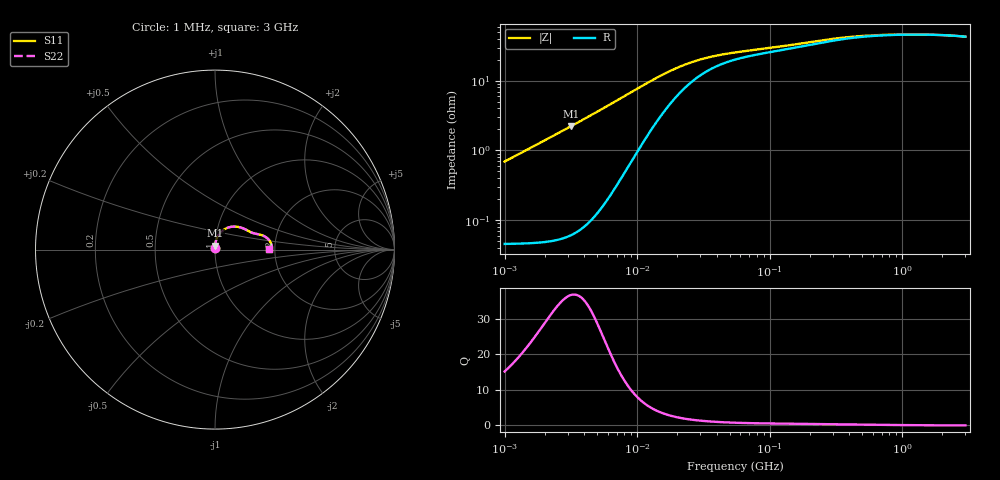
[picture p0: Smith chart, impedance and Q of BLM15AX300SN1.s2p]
! BLM15AX300SN1
# Hz S RI R 50
!Freq.(Hz) S11(Real) S11(Imag) S21(Real) S21(Imag) S12(Real) S12(Imag) S22(Real) S22(Imag)
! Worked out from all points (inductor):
!   401 points, 1 MHz to 3 GHz, reference 50 ohm
!   read as one part in series: L = 110 nH near 1.041 MHz
!   highest Q = 36.7 at 3.193 MHz (marker M1), where L = 112 nH
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1000000  0.000502 0.0069  0.9995 -0.0069  0.9995 -0.0069  0.000502 0.0069
1040844  0.000506 0.00718  0.9995 -0.00718  0.9995 -0.00718  0.000506 0.00718
1173660  0.000522 0.0081  0.9995 -0.0081  0.9995 -0.0081  0.000522 0.0081
3192880  0.00111 0.0224  0.9989 -0.0224  0.9989 -0.0224  0.00111 0.0224
3823119  0.00148 0.027  0.9985 -0.027  0.9985 -0.027  0.00148 0.027
5938264  0.00378 0.0429  0.9962 -0.0429  0.9962 -0.0429  0.00378 0.0429
8686058  0.0102 0.0643  0.9898 -0.0643  0.9898 -0.0643  0.0102 0.0643
1.172775e7  0.0228 0.0865  0.9772 -0.0865  0.9772 -0.0865  0.0228 0.0865
1.461624e7  0.0391 0.1038  0.9609 -0.1038  0.9609 -0.1038  0.0391 0.1038
1.71545e7  0.0552 0.1148  0.9448 -0.1148  0.9448 -0.1148  0.0552 0.1148
1.973457e7  0.0718 0.1222  0.9282 -0.1222  0.9282 -0.1222  0.0718 0.1222
2.270269e7  0.0897 0.1268  0.9103 -0.1268  0.9103 -0.1268  0.0897 0.1268
2.664524e7  0.1106 0.1282  0.8894 -0.1282  0.8894 -0.1282  0.1106 0.1282
3.670325e7  0.1479 0.1216  0.8521 -0.1216  0.8521 -0.1216  0.1479 0.1216
5.477226e7  0.1813 0.1065  0.8187 -0.1065  0.8187 -0.1065  0.1813 0.1065
8.854986e7  0.2086 0.0931  0.7914 -0.0931  0.7914 -0.0931  0.2086 0.0931
2.094008e8  0.2583 0.0814  0.7417 -0.0814  0.7417 -0.0814  0.2583 0.0814
2.942768e8  0.2791 0.0721  0.7209 -0.0721  0.7209 -0.0721  0.2791 0.0721
4.0536e8  0.295 0.0599  0.705 -0.0599  0.705 -0.0599  0.295 0.0599
8.005644e8  0.313 0.0326  0.687 -0.0326  0.687 -0.0326  0.313 0.0326
1.645649e9  0.314 0.0115  0.686 -0.0115  0.686 -0.0115  0.314 0.0115
3e9  0.3003 0.00232  0.6997 -0.00232  0.6997 -0.00232  0.3003 0.00232
